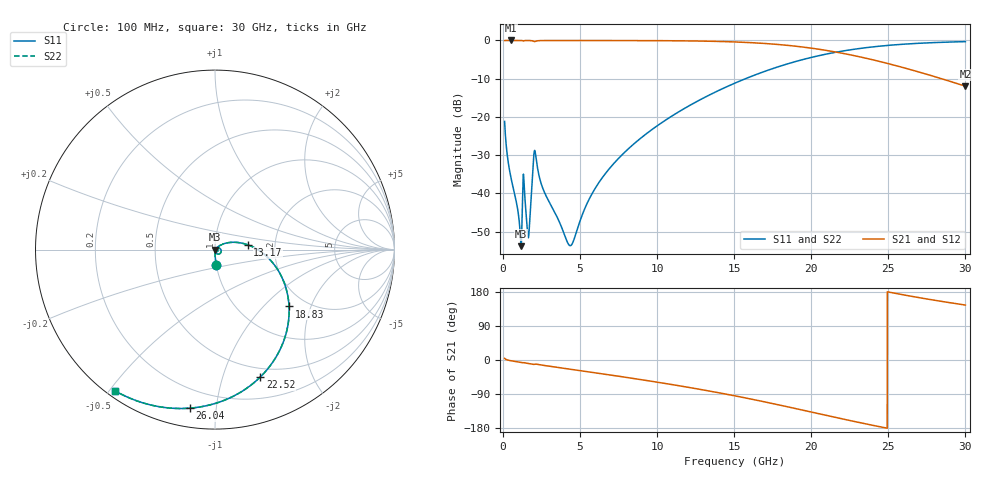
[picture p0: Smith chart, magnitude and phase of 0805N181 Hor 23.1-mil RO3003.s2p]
# GHz S MA R 50
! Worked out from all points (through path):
!   3201 points, 100 MHz to 30 GHz, reference 50 ohm
!   highest |S21| = -0.01 dB at 511.1 MHz (marker M1); lowest = -12.0 dB at 30 GHz (marker M2)
!   group delay of S21, straight-line fit = 20.9 ps
!   lowest |S11| = -53.8 dB at 1.175 GHz (marker M3), VSWR 1.00, Z = 50.2 - j0.0899 ohm
!   |S11| at or under -10 dB: start of sweep to 15.73 GHz
!   |S22| runs from -53.8 to -0.3 dB; largest |S21 - S12| = 0
!   S11 on the Smith chart (normalised r, x): 100 MHz: 1.00, -0.18; 13.17 GHz: 1.44, +0.08; 18.83 GHz: 1.64, -1.42; 22.52 GHz: 0.41, -1.33; 26.04 GHz: 0.10, -0.85; 30 GHz: 0.02, -0.52
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0.1  0.0874 -85.4  0.9959 4.5  0.9959 4.5  0.0874 -85.4
0.511125  0.0161 -90.0  0.9993 -2.0  0.9993 -2.0  0.0161 -90.0
1.07175  0.003868 -79.0  0.9988 -5.8  0.9988 -5.8  0.003868 -79.0
1.174531  0.002047 -26.0  0.998 -6.6  0.998 -6.6  0.002047 -26.0
1.389438  0.01084 -67.1  0.9944 -7.3  0.9944 -7.3  0.01084 -67.1
1.566969  0.003455 -55.9  0.9976 -8.7  0.9976 -8.7  0.003455 -55.9
1.66975  0.002872 1.1  0.9971 -9.4  0.9971 -9.4  0.002872 1.1
1.950063  0.02398 20.8  0.9796 -11.7  0.9796 -11.7  0.02398 20.8
2.090219  0.03439 -42.9  0.9707 -10.7  0.9707 -10.7  0.03439 -42.9
2.604125  0.01132 -87.0  0.9965 -14.0  0.9965 -14.0  0.01132 -87.0
4.248625  0.002162 -40.3  0.9978 -23.7  0.9978 -23.7  0.002162 -40.3
5.089563  0.00495 35.8  0.9977 -28.5  0.9977 -28.5  0.00495 35.8
6.911594  0.02127 44.1  0.9971 -39.3  0.9971 -39.3  0.02127 44.1
10.06978  0.07833 28.7  0.9934 -58.9  0.9934 -58.9  0.07833 28.7
13.17191  0.184 8.4  0.9784 -80.3  0.9784 -80.3  0.184 8.4
15.05  0.2771 -5.6  0.9555 -94.6  0.9555 -94.6  0.2771 -5.6
18.83422  0.52 -37.5  0.8472 -126.8  0.8472 -126.8  0.52 -37.5
20.03956  0.6022 -48.3  0.7909 -137.7  0.7909 -137.7  0.6022 -48.3
22.525  0.7537 -70.5  0.6488 -159.9  0.6488 -159.9  0.7537 -70.5
25.01978  0.8629 -91.2  0.4961 179.3  0.4961 179.3  0.8629 -91.2
26.03825  0.8945 -99.0  0.4375 171.5  0.4375 171.5  0.8945 -99.0
30  0.9645 -125.5  0.2523 145.0  0.2523 145.0  0.9645 -125.5
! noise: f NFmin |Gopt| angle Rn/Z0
0.1  0.0003689  0.8387  0.6406  0.0004842
3.417  0.006489  0.7109  19.13  0.004304
6.743  0.009667  0.6406  37.08  0.004592
10.06  0.01337  0.627  53.9  0.005408
13.39  0.01761  0.6342  69.52  0.006261
16.7  0.02278  0.6552  83.92  0.007205
20.03  0.02952  0.6873  97.41  0.008341
23.35  0.03881  0.7289  110.3  0.009781
26.67  0.05258  0.7781  123  0.01164
30  0.07448  0.8312  135.7  0.01391
